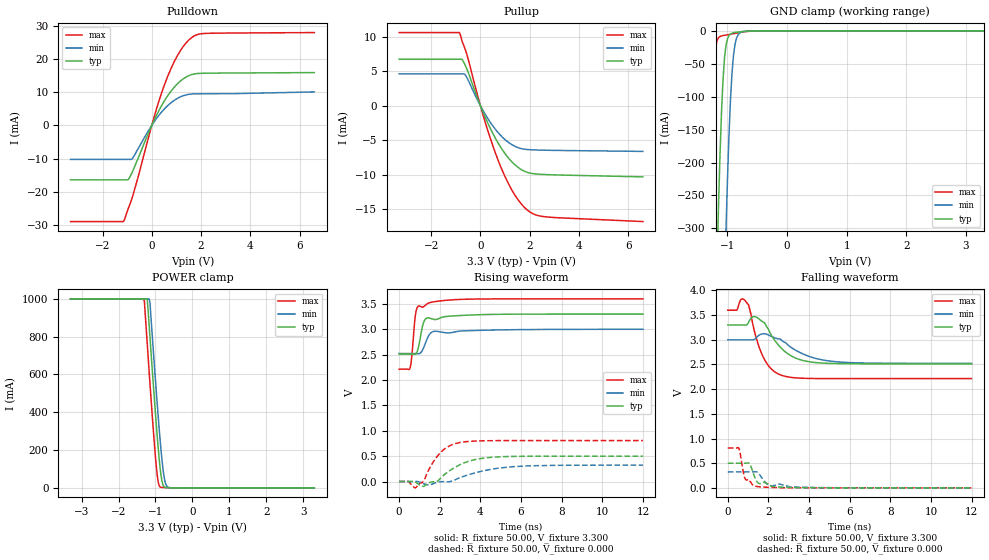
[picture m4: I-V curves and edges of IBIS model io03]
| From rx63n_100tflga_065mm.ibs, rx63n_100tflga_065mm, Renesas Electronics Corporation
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[Model]   io03
Model_type   I/O
Polarity   Non-Inverting
Enable   Active-High
Vinl  =   0.660V
Vinh  =   2.640V
Vmeas =   1.650V
Cref  =   30.00pF
| variable   typ   min   max
C_comp   4.970pF   4.970pF   4.970pF
| variable   typ   min   max
[Temperature Range]   45.000   105.000   -40.000
| variable   typ   min   max
[Voltage Range]   3.300V   3.000V   3.600V
| variable   typ   min   max
[Pullup Reference]   3.300V   3.000V   3.600V
| variable   typ   min   max
[Pulldown Reference]   0.000V   0.000V   0.000V
| variable   typ   min   max
[POWER Clamp Reference] 3.300V   3.000V   3.600V
| variable   typ   min   max
[GND Clamp Reference]   0.000V   0.000V   0.000V
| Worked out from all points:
|   slope of the pulldown table from 0 to 0.495 V, typ, clamps not added: 68.9 ohm
|   slope of the pullup table from 0 to 0.495 V, typ, clamps not added: 125 ohm
|   GND clamp passes 1 mA (typ) near -0.73 V on its own axis
|   POWER clamp passes 1 mA (typ) near -0.68 V on its own axis
|   rising waveform, R_fixture 50.00, V_fixture 3.300: 20-80 % time 250ps typ, 321ps min, 190ps max; typ from 2.51 V to 3.3 V
|   rising waveform, R_fixture 50.00, V_fixture 0.000: 20-80 % time 1.31ns typ, 1.89ns min, 877ps max; typ from 0 V to 0.499 V
|   falling waveform, R_fixture 50.00, V_fixture 3.300: 20-80 % time 1.06ns typ, 1.44ns min, 744ps max; typ from 3.3 V to 2.51 V
|   falling waveform, R_fixture 50.00, V_fixture 0.000: 20-80 % time 325ps typ, 403ps min, 271ps max; typ from 0.499 V to 0 V
[Pulldown]
| io03 Pulldown rx631_rx63n
| Thu Mar 22 17:15:49 2012
| voltage   I(typ)   I(min)   I(max)
-3.3V     -16.41mA   -10.24mA   -28.98mA
-1.15V    -16.41mA   -10.24mA   -28.98mA
-950mV    -16.26mA   -10.24mA   -24.98mA
-775mV    -13.8mA    -9.865mA   -21.27mA
100mV     1.632mA    1.118mA    2.657mA
525mV     7.544mA    5.064mA    12.43mA
800mV     10.5mA     6.935mA    17.45mA
1.075V    12.77mA    8.279mA    21.46mA
1.6V      15.26mA    9.436mA    26.34mA
1.85V     15.63mA    9.509mA    27.37mA
2.2V      15.73mA    9.534mA    27.72mA
6.6V      15.91mA    10.09mA    27.97mA
[Pullup]
| io03 Pullup rx631_rx63n
| Thu Mar 22 17:15:49 2012
| voltage   I(typ)   I(min)   I(max)
-3.3V     6.712mA    4.6mA      10.58mA
-850mV    6.712mA    4.6mA      10.58mA
-750mV    6.712mA    4.6mA      9.37mA
-600mV    5.722mA    4.374mA    7.966mA
150mV     -1.303mA   -968uA     -1.858mA
700mV     -5.288mA   -3.817mA   -7.715mA
1.3V      -8.205mA   -5.688mA   -12.35mA
1.6V      -9.105mA   -6.154mA   -13.95mA
1.925V    -9.669mA   -6.351mA   -15.16mA
2.25V     -9.879mA   -6.41mA    -15.81mA
2.7V      -9.976mA   -6.451mA   -16.1mA
6.6V      -10.3mA    -6.617mA   -16.77mA
[GND Clamp]
| io03 GNDClamp rx631_rx63n
| Thu Mar 22 17:15:49 2012
| voltage   I(typ)   I(min)   I(max)
-3.3V     -1A        -1A        -1A
-1.325V   -984.6mA   -1A        -343mA
-1.225V   -545.9mA   -1A        -51.66mA
-1.175V   -350.6mA   -894.5mA   -14.69mA
-1.15V    -263.6mA   -785.8mA   -10.32mA
-1.125V   -186.6mA   -680mA     -8.582mA
-1.075V   -73.84mA   -479.8mA   -7.226mA
-1.025V   -22.04mA   -301.7mA   -6.404mA
-975mV    -7.162mA   -158.6mA   -5.611mA
-925mV    -3.609mA   -64.96mA   -4.78mA
-800mV    -1.61mA    -3.681mA   -2.675mA
3.3V      0A         0A         0A
[POWER Clamp]
| io03 PWRClamp rx631_rx63n
| Thu Mar 22 17:15:49 2012
| voltage   I(typ)   I(min)   I(max)
-3.3V     1A         1A         1A
-1.325V   1A         1A         1A
-1.3V     1A         1A         986.2mA
-1.225V   1A         1A         768.5mA
-1.15V    800.7mA    982mA      555.2mA
-975mV    328.6mA    502.4mA    107.8mA
-925mV    209mA      374.7mA    29.63mA
-875mV    106.7mA    255.4mA    5.038mA
-825mV    36.52mA    149.8mA    2.269mA
-775mV    8.064mA    68.01mA    1.837mA
-650mV    739uA      2.543mA    864uA
3.3V      0A         0A         0A
[Ramp]
dV/dt_r   0.300/1.31n   0.193/1.89n   0.484/876.03p
dV/dt_f   0.473/1.06n   0.286/1.44n   0.832/745.27p
R_load = 50.00ohm
[Rising Waveform]
| io03 Rising-High rx631_rx63n
| Thu Mar 22 17:15:49 2012
R_fixture = 50.00
V_fixture = 3.300
V_fixture_min = 3.000
V_fixture_max = 3.600
C_fixture = 0.00pF
| Time   V(typ)   V(min)   V(max)
0s        2.512V     2.523V     2.214V
540ps     2.512V     2.523V     2.241V
625ps     2.513V     2.523V     2.477V
785ps     2.507V     2.523V     3.229V
890ps     2.563V     2.52V      3.429V
1.06ns    2.875V     2.539V     3.449V
1.22ns    3.15V      2.652V     3.45V
1.53ns    3.217V     2.917V     3.528V
3.845ns   3.286V     2.978V     3.597V
12ns      3.3V       3V         3.6V
[Rising Waveform]
| io03 Rising-Low rx631_rx63n
| Thu Mar 22 17:15:49 2012
R_fixture = 50.00
V_fixture = 0.000
C_fixture = 0.00pF
| Time   V(typ)   V(min)   V(max)
0s        0V         0V         0V
465ps     0V         0V         -1mV
810ps     -12mV      1mV        -123mV
1.2ns     -96mV      -43mV      5mV
1.575ns   -11mV      -59mV      317mV
2.07ns    80mV       -4mV       584mV
3.07ns    345mV      88mV       774mV
4.09ns    457mV      205mV      802mV
5.82ns    496mV      297mV      806mV
12ns      499mV      322mV      807mV
[Falling Waveform]
| io03 Falling-High rx631_rx63n
| Thu Mar 22 17:15:49 2012
R_fixture = 50.00
V_fixture = 3.300
V_fixture_min = 3.000
V_fixture_max = 3.600
C_fixture = 0.00pF
| Time   V(typ)   V(min)   V(max)
0s        3.3V       3V         3.6V
440ps     3.3V       3V         3.601V
865ps     3.299V     3V         3.79V
1.04ns    3.368V     3V         3.687V
1.275ns   3.471V     3.002V     3.238V
1.795ns   3.351V     3.122V     2.611V
2.775ns   2.776V     2.954V     2.265V
3.79ns    2.572V     2.698V     2.22V
5.185ns   2.52V      2.562V     2.214V
12ns      2.512V     2.523V     2.214V
[Falling Waveform]
| io03 Falling-Low rx631_rx63n
| Thu Mar 22 17:15:49 2012
R_fixture = 50.00
V_fixture = 0.000
C_fixture = 0.00pF
| Time   V(typ)   V(min)   V(max)
0s        499mV      322mV      807mV
530ps     499mV      322mV      810mV
595ps     499mV      322mV      732mV
775ps     499mV      322mV      299mV
855ps     499mV      322mV      185mV
1.085ns   481mV      322mV      134mV
1.43ns    130mV      321mV      28mV
1.89ns    91mV       94mV       12mV
2.14ns    35mV       44mV       8mV
12ns      0V         0V         0V
